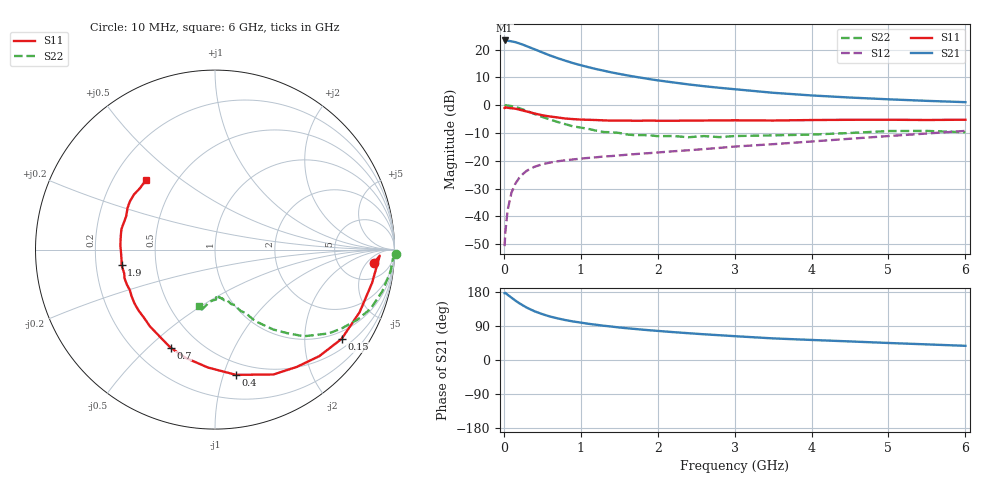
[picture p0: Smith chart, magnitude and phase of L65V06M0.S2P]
!  INFINEON TECHNOLOGIES Small Signal Semiconductors
! BFR380L3 , Si-NPN RF-Transistor in TSLP-3-1
!  Vce=5 V,  Ic=6 mA
! Common Emitter S-Parameters:  07. March 2005
#  GHz  S  MA  R  50
! f  S11  S21  S12  S22
! GHz  Mag  Ang  Mag  Ang  Mag  Ang  Mag  Ang
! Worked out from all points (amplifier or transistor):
!   36 points, 10 MHz to 6 GHz, reference 50 ohm
!   highest |S21| = 23.3 dB at 10 MHz (marker M1)
!   |S21| within 3 dB of that: start of sweep to 383.4 MHz
!   unconditionally stable (mu >= 1): 2.67 GHz to 4.581 GHz
!   at 250 MHz: K = 0.17, MSG = 23.2 dB, |S12| = -24.7 dB
!   at 1.4 GHz: K = 0.75, MSG = 15.0 dB, |S12| = -18.3 dB
!   at 6 GHz: K = 0.93, MSG = 5.2 dB, |S12| = -9.3 dB
!   S11 on the Smith chart (normalised r, x): 10 MHz: 11, -8; 150 MHz: 0.76, -2.98; 400 MHz: 0.39, -1.10; 700 MHz: 0.34, -0.59; 1.9 GHz: 0.31, -0.07; 6 GHz: 0.34, +0.38
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0.01  0.888 -4.8  14.58 176.5  0.0029 83.6  1.011 -1.5
0.02  0.9185 -2.1  14.48 177.1  0.0053 87.8  0.9922 -3.0
0.05  0.8946 -12.0  14.42 172.0  0.0131 84.9  0.9855 -7.1
0.1  0.8779 -23.4  14.04 164.4  0.0268 79.3  0.9604 -14.1
0.15  0.8631 -35.2  13.59 156.8  0.0387 71.8  0.9276 -20.8
0.2  0.8307 -45.6  12.91 149.9  0.0491 68.6  0.8848 -26.2
0.25  0.7967 -55.1  12.21 143.9  0.0581 62.9  0.8321 -31.8
0.3  0.7683 -64.9  11.46 138.0  0.0663 59.4  0.7872 -36.4
0.4  0.7075 -80.5  10.11 128.5  0.078 53.4  0.6914 -44.3
0.5  0.658 -93.5  8.884 121.1  0.0863 49.3  0.6135 -49.3
0.6  0.6247 -105.3  7.83 114.7  0.0925 46.4  0.5509 -53.9
0.7  0.5999 -114.4  6.998 109.8  0.0977 45.0  0.4976 -57.4
0.9  0.5606 -130.4  5.705 101.7  0.1053 43.1  0.4149 -62.9
1.1  0.5445 -141.4  4.814 95.5  0.1124 43.1  0.3736 -67.0
1.5  0.5284 -158.5  3.653 85.8  0.1247 44.9  0.3161 -73.5
1.9  0.5275 -170.7  2.93 78.4  0.1372 47.5  0.2866 -79.8
2.2  0.5236 -177.5  2.564 73.6  0.1477 49.5  0.2785 -81.4
2.8  0.5314 170.3  2.053 65.4  0.1701 53.7  0.2658 -88.6
3.5  0.5285 159.5  1.669 57.0  0.1985 56.0  0.2858 -93.8
4.5  0.5447 150.8  1.37 49.0  0.2485 59.6  0.3154 -99.2
5.5  0.5402 140.6  1.194 41.2  0.3088 59.9  0.3434 -104.2
6  0.5468 134.5  1.131 37.4  0.3438 59.0  0.3257 -106.3
